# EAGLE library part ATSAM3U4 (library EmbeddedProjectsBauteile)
Atmel AT91SAM ARM-based Flash MCU, SAM3U Series
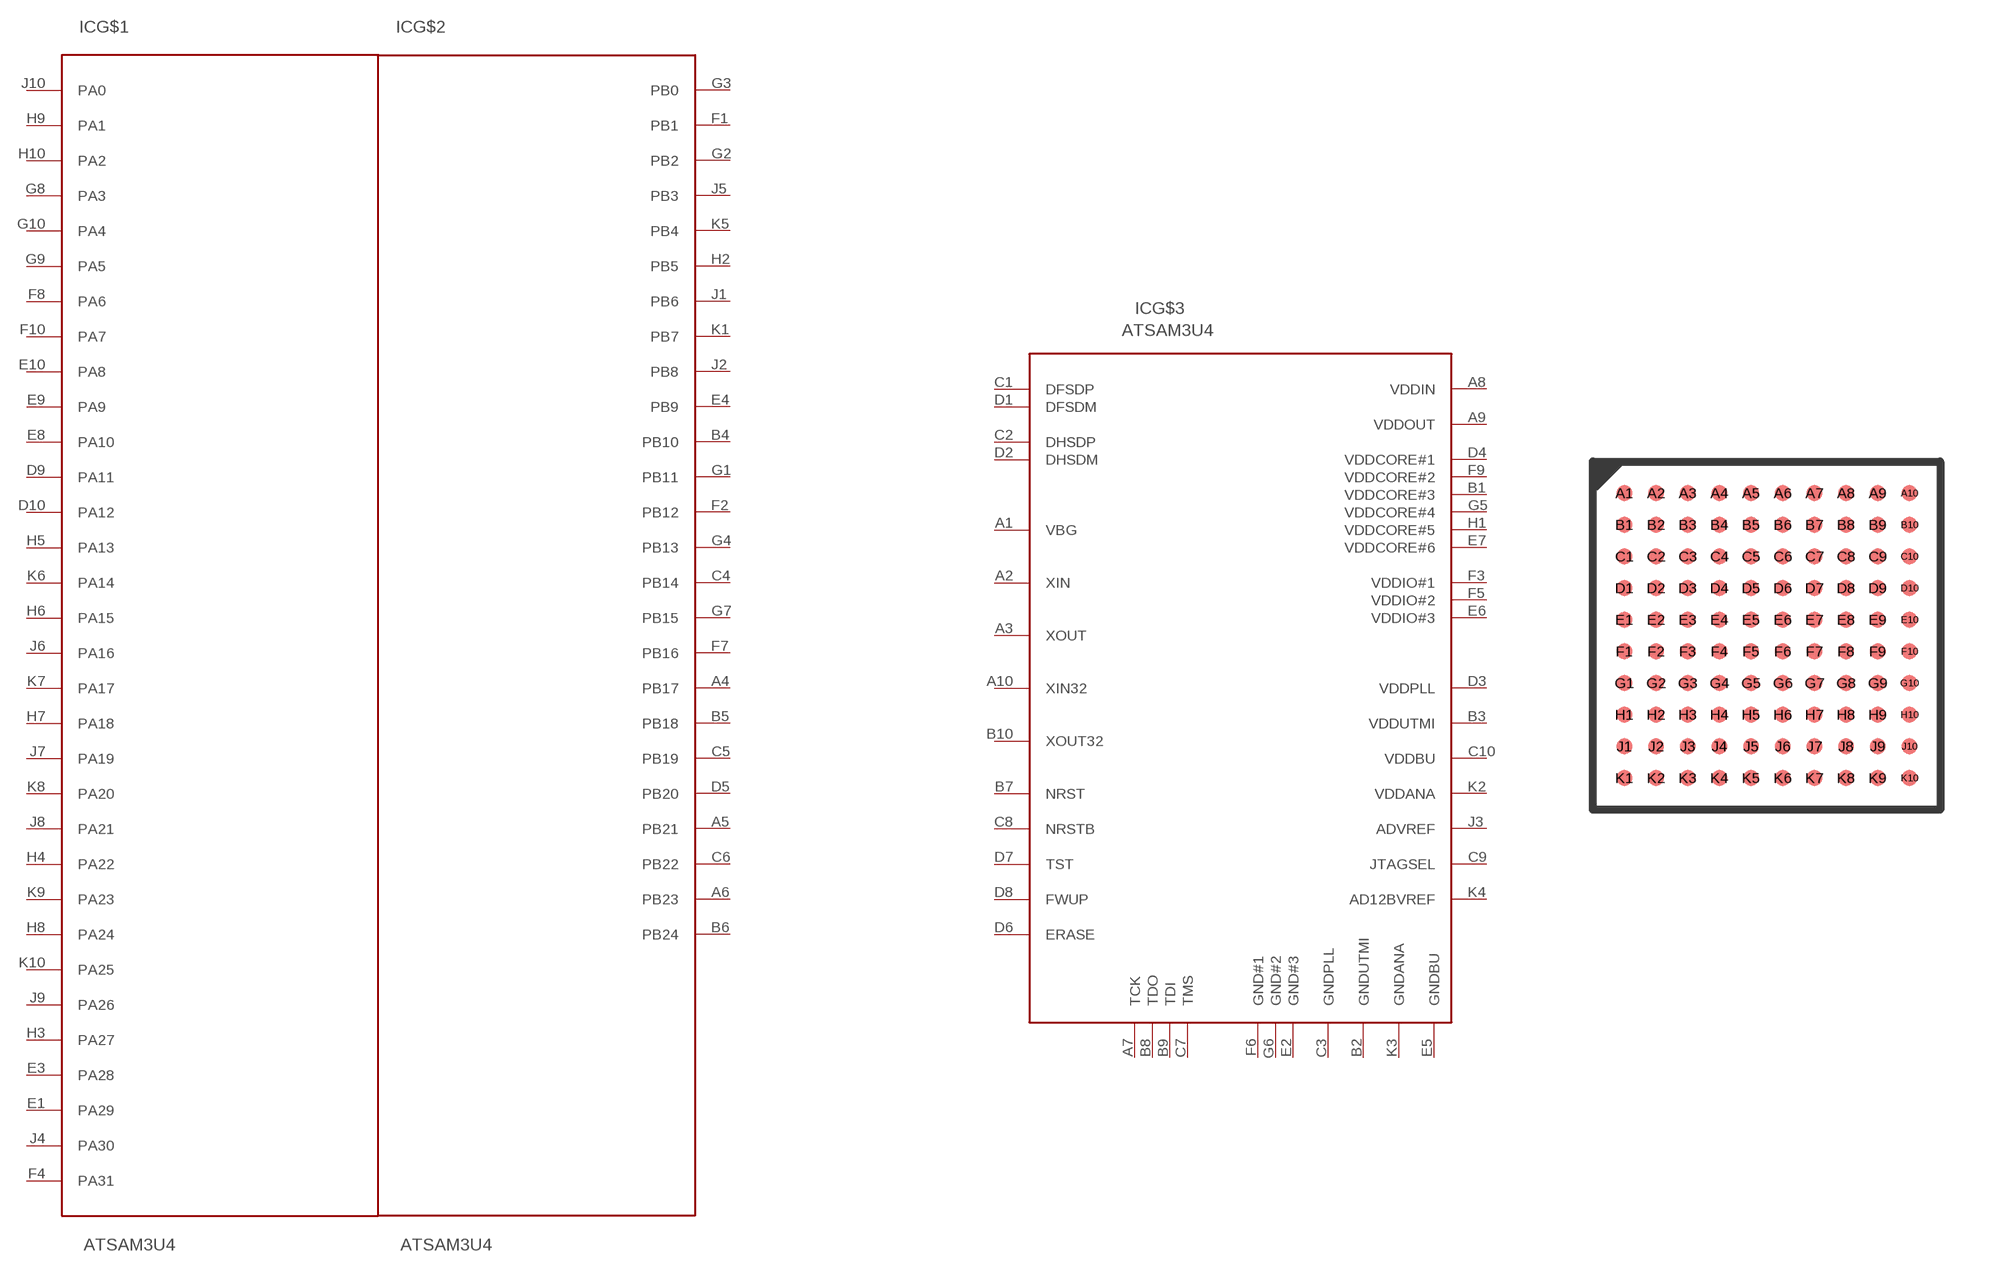
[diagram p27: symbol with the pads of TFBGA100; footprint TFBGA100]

Designator prefix IC; gates G$1=SAM3_PA G$2=SAM3_PB G$3=SAM3_PWR

## ATSAM3U4 (EP: 401038)  [TFBGA100]
A1  G$3:VBG
A2  G$3:XIN  in
A3  G$3:XOUT  out
A4  G$2:PB17
A5  G$2:PB21
A6  G$2:PB23
A7  G$3:TCK
A8  G$3:VDDIN  pwr
A9  G$3:VDDOUT  pwr
A10  G$3:XIN32  in
B1  G$3:VDDCORE#3  pwr
B2  G$3:GNDUTMI  pwr
B3  G$3:VDDUTMI  pwr
B4  G$2:PB10
B5  G$2:PB18
B6  G$2:PB24
B7  G$3:NRST  in
B8  G$3:TDO
B9  G$3:TDI
B10  G$3:XOUT32  out
C1  G$3:DFSDP
C2  G$3:DHSDP
C3  G$3:GNDPLL  pwr
C4  G$2:PB14
C5  G$2:PB19
C6  G$2:PB22
C7  G$3:TMS
C8  G$3:NRSTB  in
C9  G$3:JTAGSEL  pwr
C10  G$3:VDDBU  pwr
D1  G$3:DFSDM
D2  G$3:DHSDM
D3  G$3:VDDPLL  pwr
D4  G$3:VDDCORE#1  pwr
D5  G$2:PB20
D6  G$3:ERASE
D7  G$3:TST
D8  G$3:FWUP  in
D9  G$1:PA11
D10  G$1:PA12
E1  G$1:PA29
E2  G$3:GND#3  pwr
E3  G$1:PA28
E4  G$2:PB9
E5  G$3:GNDBU  pwr
E6  G$3:VDDIO#3  pwr
E7  G$3:VDDCORE#6  pwr
E8  G$1:PA10
E9  G$1:PA9
E10  G$1:PA8
F1  G$2:PB1
F2  G$2:PB12
F3  G$3:VDDIO#1  pwr
F4  G$1:PA31
F5  G$3:VDDIO#2  pwr
F6  G$3:GND#1  pwr
F7  G$2:PB16
F8  G$1:PA6
F9  G$3:VDDCORE#2  pwr
F10  G$1:PA7
G1  G$2:PB11
G2  G$2:PB2
G3  G$2:PB0
G4  G$2:PB13
G5  G$3:VDDCORE#4  pwr
G6  G$3:GND#2  pwr
G7  G$2:PB15
G8  G$1:PA3
G9  G$1:PA5
G10  G$1:PA4
H1  G$3:VDDCORE#5  pwr
H2  G$2:PB5
H3  G$1:PA27
H4  G$1:PA22
H5  G$1:PA13
H6  G$1:PA15
H7  G$1:PA18
H8  G$1:PA24
H9  G$1:PA1
H10  G$1:PA2
J1  G$2:PB6
J2  G$2:PB8
J3  G$3:ADVREF  pwr
J4  G$1:PA30
J5  G$2:PB3
J6  G$1:PA16
J7  G$1:PA19
J8  G$1:PA21
J9  G$1:PA26
J10  G$1:PA0
K1  G$2:PB7
K2  G$3:VDDANA  pwr
K3  G$3:GNDANA  pwr
K4  G$3:AD12BVREF  pwr
K5  G$2:PB4
K6  G$1:PA14
K7  G$1:PA17
K8  G$1:PA20
K9  G$1:PA23
K10  G$1:PA25

## Footprint TFBGA100 (pad centres in mm)
smd 0.399 x 0.399: A1 -3.6,3.6; A2 -2.8,3.6; A3 -2,3.6; A4 -1.2,3.6; A5 -0.4,3.6; A6 0.4,3.6; A7 1.2,3.6; A8 2,3.6; A9 2.8,3.6; A10 3.6,3.6; B1 -3.6,2.8; B2 -2.8,2.8; B3 -2,2.8; B4 -1.2,2.8; B5 -0.4,2.8; B6 0.4,2.8; B7 1.2,2.8; B8 2,2.8; B9 2.8,2.8; B10 3.6,2.8; C1 -3.6,2; C2 -2.8,2; C3 -2,2; C4 -1.2,2; C5 -0.4,2; C6 0.4,2; C7 1.2,2; C8 2,2; C9 2.8,2; C10 3.6,2; D1 -3.6,1.2; D2 -2.8,1.2; D3 -2,1.2; D4 -1.2,1.2; D5 -0.4,1.2; D6 0.4,1.2; D7 1.2,1.2; D8 2,1.2; D9 2.8,1.2; D10 3.6,1.2; E1 -3.6,0.4; E2 -2.8,0.4; E3 -2,0.4; E4 -1.2,0.4; E5 -0.4,0.4; E6 0.4,0.4; E7 1.2,0.4; E8 2,0.4; E9 2.8,0.4; E10 3.6,0.4; F1 -3.6,-0.4; F2 -2.8,-0.4; F3 -2,-0.4; F4 -1.2,-0.4; F5 -0.4,-0.4; F6 0.4,-0.4; F7 1.2,-0.4; F8 2,-0.4; F9 2.8,-0.4; F10 3.6,-0.4; G1 -3.6,-1.2; G2 -2.8,-1.2; G3 -2,-1.2; G4 -1.2,-1.2; G5 -0.4,-1.2; G6 0.4,-1.2; G7 1.2,-1.2; G8 2,-1.2; G9 2.8,-1.2; G10 3.6,-1.2; H1 -3.6,-2; H2 -2.8,-2; H3 -2,-2; H4 -1.2,-2; H5 -0.4,-2; H6 0.4,-2; H7 1.2,-2; H8 2,-2; H9 2.8,-2; H10 3.6,-2; J1 -3.6,-2.8; J2 -2.8,-2.8; J3 -2,-2.8; J4 -1.2,-2.8; J5 -0.4,-2.8; J6 0.4,-2.8; J7 1.2,-2.8; J8 2,-2.8; J9 2.8,-2.8; J10 3.6,-2.8; K1 -3.6,-3.6; K2 -2.8,-3.6; K3 -2,-3.6; K4 -1.2,-3.6; K5 -0.4,-3.6; K6 0.4,-3.6; K7 1.2,-3.6; K8 2,-3.6; K9 2.8,-3.6; K10 3.6,-3.6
